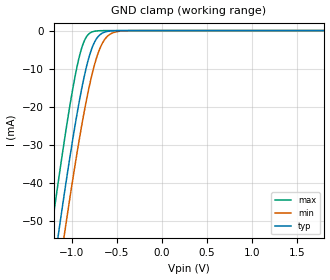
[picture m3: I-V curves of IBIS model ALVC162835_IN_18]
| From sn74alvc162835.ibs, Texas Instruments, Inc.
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[Model]   ALVC162835_IN_18
Model_type  Input
Vinl=0.5775
Vinh=1.2675
| variable   typ   min   max
C_comp   10.83pF   10.58pF   10.95pF
[Temperature Range]   40   100   -40
| Ambient temperature   25   85   -40
[Voltage range]   1.8   1.65   1.95
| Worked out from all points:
|   GND clamp passes 1 mA (typ) near -0.68 V on its own axis
[GND Clamp]
| ALVC162835_IN_18
|   Voltage   I(typ)   I(min)   I(max)
-1.8V     -169.5mA   -179.7mA   -156.7mA
-1.245V   -70.18mA   -81.02mA   -56.25mA
-1.22V    -65.92mA   -76.78mA   -51.96mA
-1.14V    -52.55mA   -63.42mA   -38.55mA
-1.075V   -42.06mA   -52.87mA   -28.16mA
-920mV    -19.37mA   -29.44mA   -7.486mA
-860mV    -12.16mA   -21.41mA   -2.808mA
-795mV    -6.112mA   -13.8mA    -645.2uA
-730mV    -2.404mA   -7.745mA   -117.8uA
-660mV    -692.8uA   -3.428mA   -17.66uA
-495mV    -25.94uA   -270.9uA   -195.5nA
1.8V      1.111nA    59.61nA    3.29pA
